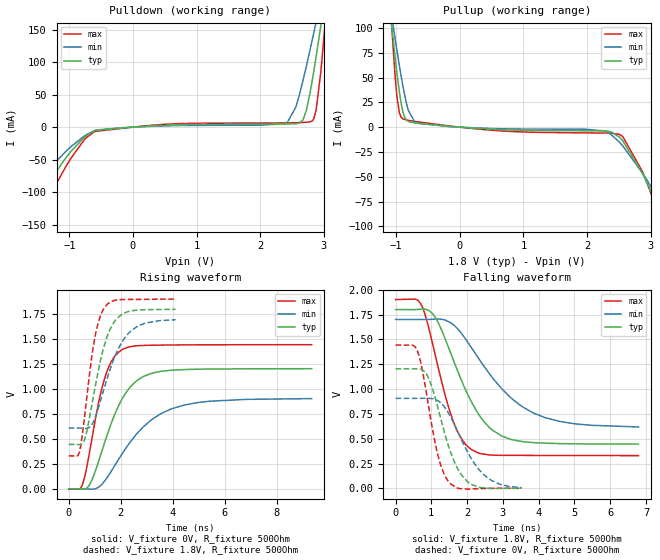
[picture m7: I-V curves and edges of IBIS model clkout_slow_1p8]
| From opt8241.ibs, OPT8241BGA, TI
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|   clkout_slow_1p8 Model
[Model]   clkout_slow_1p8
Model_type   Output
Polarity   Non-Inverting
Vmeas = 0.9
Vref  = 0
Cref  = 2pF
Rref  = 500
|   typ   min   max
|   (nom PVT)   (fast PVT)   (slow PVT)
C_comp   2.233e-12   2.012e-12   2.445e-12
| Where nom  PVT is Nominal Process, 1.8V, 27C
|   Fast PVT is Strong Process,  1.9V, -40C
|   Slow PVT is Weak Process,   1.7V, 125C
[Voltage Range]   1.8   1.7   1.9
|Junction Temperature
[Temperature Range]   27   125   -40
[Pullup Reference]   1.8   1.7   1.9
[Pulldown Reference]   0   0   0
[Power Clamp Reference]   1.8   1.7   1.9
[GND Clamp Reference]   0   0   0
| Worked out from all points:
|   slope of the pulldown table from 0 to 0.27 V, typ, clamps not added: 150 ohm
|   slope of the pullup table from 0 to 0.27 V, typ, clamps not added: 218 ohm
|   falling waveform, V_fixture 1.8V, R_fixture 500Ohm: 20-80 % time 1.02ns typ, 1.5ns min, 695ps max; typ from 1.8 V to 0.446 V
|   rising waveform, V_fixture 0V, R_fixture 500Ohm: 20-80 % time 1.1ns typ, 1.72ns min, 695ps max; typ from 0 V to 1.2 V
|   rising waveform, V_fixture 1.8V, R_fixture 500Ohm: 20-80 % time 679ps typ, 908ps min, 489ps max; typ from 0.444 V to 1.8 V
|   falling waveform, V_fixture 0V, R_fixture 500Ohm: 20-80 % time 609ps typ, 810ps min, 451ps max; typ from 1.2 V to 0.001 V
[Pulldown]
|   Voltage   I(typ)   I(min)   I(max)
-1.8V     -251.1mA   -143.5mA   -360.3mA
-1.654V   -148mA     -101.6mA   -228.5mA
-1.551V   -118.3mA   -89.17mA   -157mA
-973.8mV  -37.41mA   -30.06mA   -47.94mA
-613.4mV  -6.144mA   -5.669mA   -7.588mA
2.416V    4.784mA    5.284mA    6.503mA
2.675V    11.32mA    72.16mA    7.22mA
2.819V    71.52mA    134mA      9.605mA
2.88V     108.5mA    161.8mA    26.12mA
2.954V    156mA      195.7mA    84.86mA
3.068V    233.1mA    248.9mA    209.3mA
3.6V      602.9mA    497mA      863mA
[Pullup]
|   Voltage   I(typ)   I(min)   I(max)
-1.8V     604.2mA    451.5mA    989.3mA
-1.067V   100.6mA    111.1mA    98.54mA
-987.4mV  54.53mA    77.46mA    30.84mA
-948.8mV  35.34mA    61.99mA    14.45mA
-895.6mV  15.9mA     42.21mA    8.501mA
-810mV    5.73mA     17.04mA    6.949mA
-698.4mV  4.153mA    4.204mA    5.681mA
2.282V    -3.804mA   -3.92mA    -5.927mA
2.51V     -10.03mA   -15.15mA   -7.304mA
3.307V    -107.7mA   -92.57mA   -119.4mA
3.397V    -123.9mA   -105.4mA   -136.8mA
3.598V    -246.4mA   -202.6mA   -264.6mA
[Ramp]
R_load = 500
|   typ   min   max
dV/dt_r   0.721328/1.09385e-09   0.542668/1.71634e-09   0.865237/6.94336e-10
dV/dt_f   0.813168/1.01739e-09   0.654487/1.52209e-09   0.942109/6.94975e-10
[Falling Waveform]
V_fixture = 1.8V
V_fixture_min = 1.7V
V_fixture_max = 1.9V
R_fixture = 500Ohm
|   Time   V(typ)   V(min)   V(max)
0s        1.8V       1.7V       1.9V
718ps     1.804V     1.7V       1.849V
1.048ns   1.753V     1.702V     1.437V
1.53ns    1.373V     1.669V     760.5mV
1.792ns   1.131V     1.582V     529.5mV
2.108ns   878.9mV    1.422V     393.7mV
2.718ns   583.1mV    1.108V     334.7mV
3.83ns    461.2mV    762.8mV    331.8mV
4.992ns   448.7mV    650.9mV    330.5mV
6.788ns   445.6mV    618.2mV    330.2mV
[Rising Waveform]
V_fixture = 0V
V_fixture_min = 0V
V_fixture_max = 0V
R_fixture = 500Ohm
|   Time   V(typ)   V(min)   V(max)
0s        2.414nV    154.5nV    1.12nV
526ps     -3.716mV   351.5uV    38.82mV
878ps     78.99mV    -3.807mV   477.3mV
1.158ns   280.2mV    16.83mV    872.3mV
1.384ns   464.1mV    77.98mV    1.106V
1.72ns    711.4mV    209.8mV    1.308V
2.046ns   896.1mV    346.1mV    1.392V
2.886ns   1.125V     624.1mV    1.435V
4.442ns   1.193V     837.8mV    1.44V
9.34ns    1.202V     902.3mV    1.442V
[Rising Waveform]
V_fixture = 1.8V
V_fixture_min = 1.7V
V_fixture_max = 1.9V
R_fixture = 500Ohm
|   Time   V(typ)   V(min)   V(max)
0s        444.1mV    607.8mV    329.2mV
414ps     442.5mV    607.7mV    366mV
656ps     531.2mV    605.2mV    822.8mV
960ps     935.9mV    675.7mV    1.443V
1.124ns   1.163V     795.6mV    1.649V
1.32ns    1.389V     966mV      1.789V
1.796ns   1.686V     1.337V     1.887V
2.366ns   1.779V     1.573V     1.895V
2.946ns   1.792V     1.659V     1.896V
4.11ns    1.796V     1.691V     1.899V
[Falling Waveform]
|Gnd
V_fixture = 0V
V_fixture_min = 0V
V_fixture_max = 0V
R_fixture = 500Ohm
|   Time   V(typ)   V(min)   V(max)
0s        1.203V     906mV      1.443V
610ps     1.204V     906mV      1.385V
732ps     1.196V     906.2mV    1.22V
892ps     1.131V     906.9mV    893mV
1.158ns   846.2mV    888.2mV    371.1mV
1.492ns   412.7mV    749.8mV    62.39mV
1.854ns   130mV      478.3mV    -3.4mV
2.364ns   8.915mV    176.1mV    -2.64mV
2.894ns   -852.6uV   44.35mV    1.453mV
3.524ns   1.451mV    7.166mV    845uV
